PROGRAM MAIN
VAR	
	nIntVar1 : INT := 15;
	pInt : POINTER TO INT;	
	pInt2 : POINTER TO INT;	
	valViaPointer : INT ;

	
	singleRowArray : ARRAY [0..MaxColumn] OF LREAL;
	singleRowPointer : POINTER TO LREAL ;
	columnVal1 : LREAL;
	columnVal2 : LREAL;
	columnVal3 : LREAL;
	add1 : POINTER TO LREAL ;
	add2 : POINTER TO LREAL ;
	add3 : POINTER TO LREAL ;
	nIntSize  : UINT;	
		
	plainInt : ARRAY[0..2] OF INT;	
	plainIntAdd0 : POINTER TO INT;
	plainIntAdd1 : POINTER TO INT;
	plainIntAdd2 : POINTER TO INT;
	plainIntPointer : POINTER TO INT;
	delta : DWORD;
	test : INT ;
	
	page 	: ARRAY[0..MaxRow]OF ARRAY[0..MaxColumn]OF REAL;	
	i : INT := 0;
	j : INT := 0;
	k: INT := 0;
	initDone : BOOL:= FALSE; 
	pageFirstRow		    : POINTER TO ARRAY[0..MaxColumn] OF REAL;
	pageSecondRow		    : POINTER TO ARRAY[0..MaxColumn] OF REAL;
	pageThirdRow		    : POINTER TO ARRAY[0..MaxColumn] OF REAL;
	nVarSize  : UINT;
	calLastIndexAddress : POINTER TO UINT;
	dataReal : REAL := 0.0;
	motorSpeed :  REAL;
	//motorSpeed :  POINTER TO REAL; // uncomment this and comment previous line to produce page fault
	fnMOTORBLOCK : MOTORBLOCK;
	
	//References
	refInt  : REFERENCE TO INT;
    nA      : INT := 200;	
END_VAR


VAR CONSTANT
MaxRow : INT := 3;
MaxColumn : INT := 5;
END_VAR

IF NOT initDone THEN
	
	FOR k := 0 TO MaxColumn DO
		singleRowArray[k]:= 3.0007 + k;
	END_FOR		
	
singleRowPointer := ADR(singleRowArray);
singleRowPointer := ADR(singleRowArray[0]);

columnVal1 := singleRowPointer^;

// Dereference index 3 (address of array and some pointer arithmetic)
singleRowPointer := ADR(singleRowArray) + 3 * SIZEOF(singleRowPointer^);
columnVal2 := singleRowPointer^;

// Dereference next index (pointer arithmetic)
singleRowPointer := singleRowPointer + SIZEOF(singleRowPointer^);
columnVal3 := singleRowPointer^;	

add1 := ADR(columnVal1);
add2 := ADR(columnVal2);
add3 := ADR(columnVal3);
nIntSize:= SIZEOF(LREAL);

	FOR i := 0 TO MaxRow DO
		FOR j := 0 TO MaxColumn DO
			page[i][j]:= 0.0;
		END_FOR	
	END_FOR
	page[0][0]:= 0;
	page[1][0]:= 10;
	page[2][0]:= 20;
	page[3][0]:= 30;
	
	page[0][1]:= 1;
	page[1][1]:= 11;
	page[2][1]:= 21;
	page[3][1]:= 31;
	
	page[0][2]:= 2;
	page[1][2]:= 12;
	page[2][2]:= 22;
	page[3][2]:= 32;	
	
	page[0][3]:= 3;
	page[1][3]:= 13;
	page[2][3]:= 23;
	page[3][3]:= 33;	

	page[0][4]:= 4;
	page[1][4]:= 14;
	page[2][4]:= 24;
	page[3][4]:= 34;	

	page[0][5]:= 5;
	page[1][5]:= 15;
	page[2][5]:= 25;
	page[3][5]:= 35;		
	
	
	initDone:= TRUE;
	pageFirstRow := ADR(page);
	pageSecondRow := ADR(page[1]);
	pageThirdRow :=ADR(page[2]);
	
	nVarSize:= SIZEOF(REAL);
	
	
	
	
	FOR j := 0 TO MaxColumn DO
		plainInt[j]:= 3 + j;
	END_FOR	
		
	plainIntAdd0:= ADR(plainInt[0]);
	plainIntAdd1:= ADR(plainInt[1]);
	
	plainIntAdd2:= plainIntAdd0 + 2 * SIZEOF (INT);
	test := plainIntAdd2^;
	plainIntAdd2^ := 321;
	delta:= plainIntAdd1-plainIntAdd0;
	calLastIndexAddress:= ADR(pageFirstRow) + nVarSize*5;
	
plainIntPointer:= ADR(plainInt) + 0 * SIZEOF (INT); //First one
plainIntPointer:= ADR(plainInt) + 1 * SIZEOF (INT); //Second one and so on
plainIntPointer:= ADR(plainInt) + 2 * SIZEOF (INT); //Third one and so on	


END_IF

pInt := ADR(nIntVar1); //pInt is the address where it was saved
valViaPointer := pInt^;
pInt2 := pInt;
pInt^:= 345;
// try to access page value at particular index, check what you get if you don't assign valid value to i and j
i:= 2;
j:= 3;
dataReal := page[i][j]; 
fnMOTORBLOCK(inputPointer := ADR(motorSpeed));
//fnMOTORBLOCK(inputPointer := motorSpeed); // uncomment this and comment previous line to produce page fault

//References
refInt REF= nA;         // refInt points now to nA

END_PROGRAM
